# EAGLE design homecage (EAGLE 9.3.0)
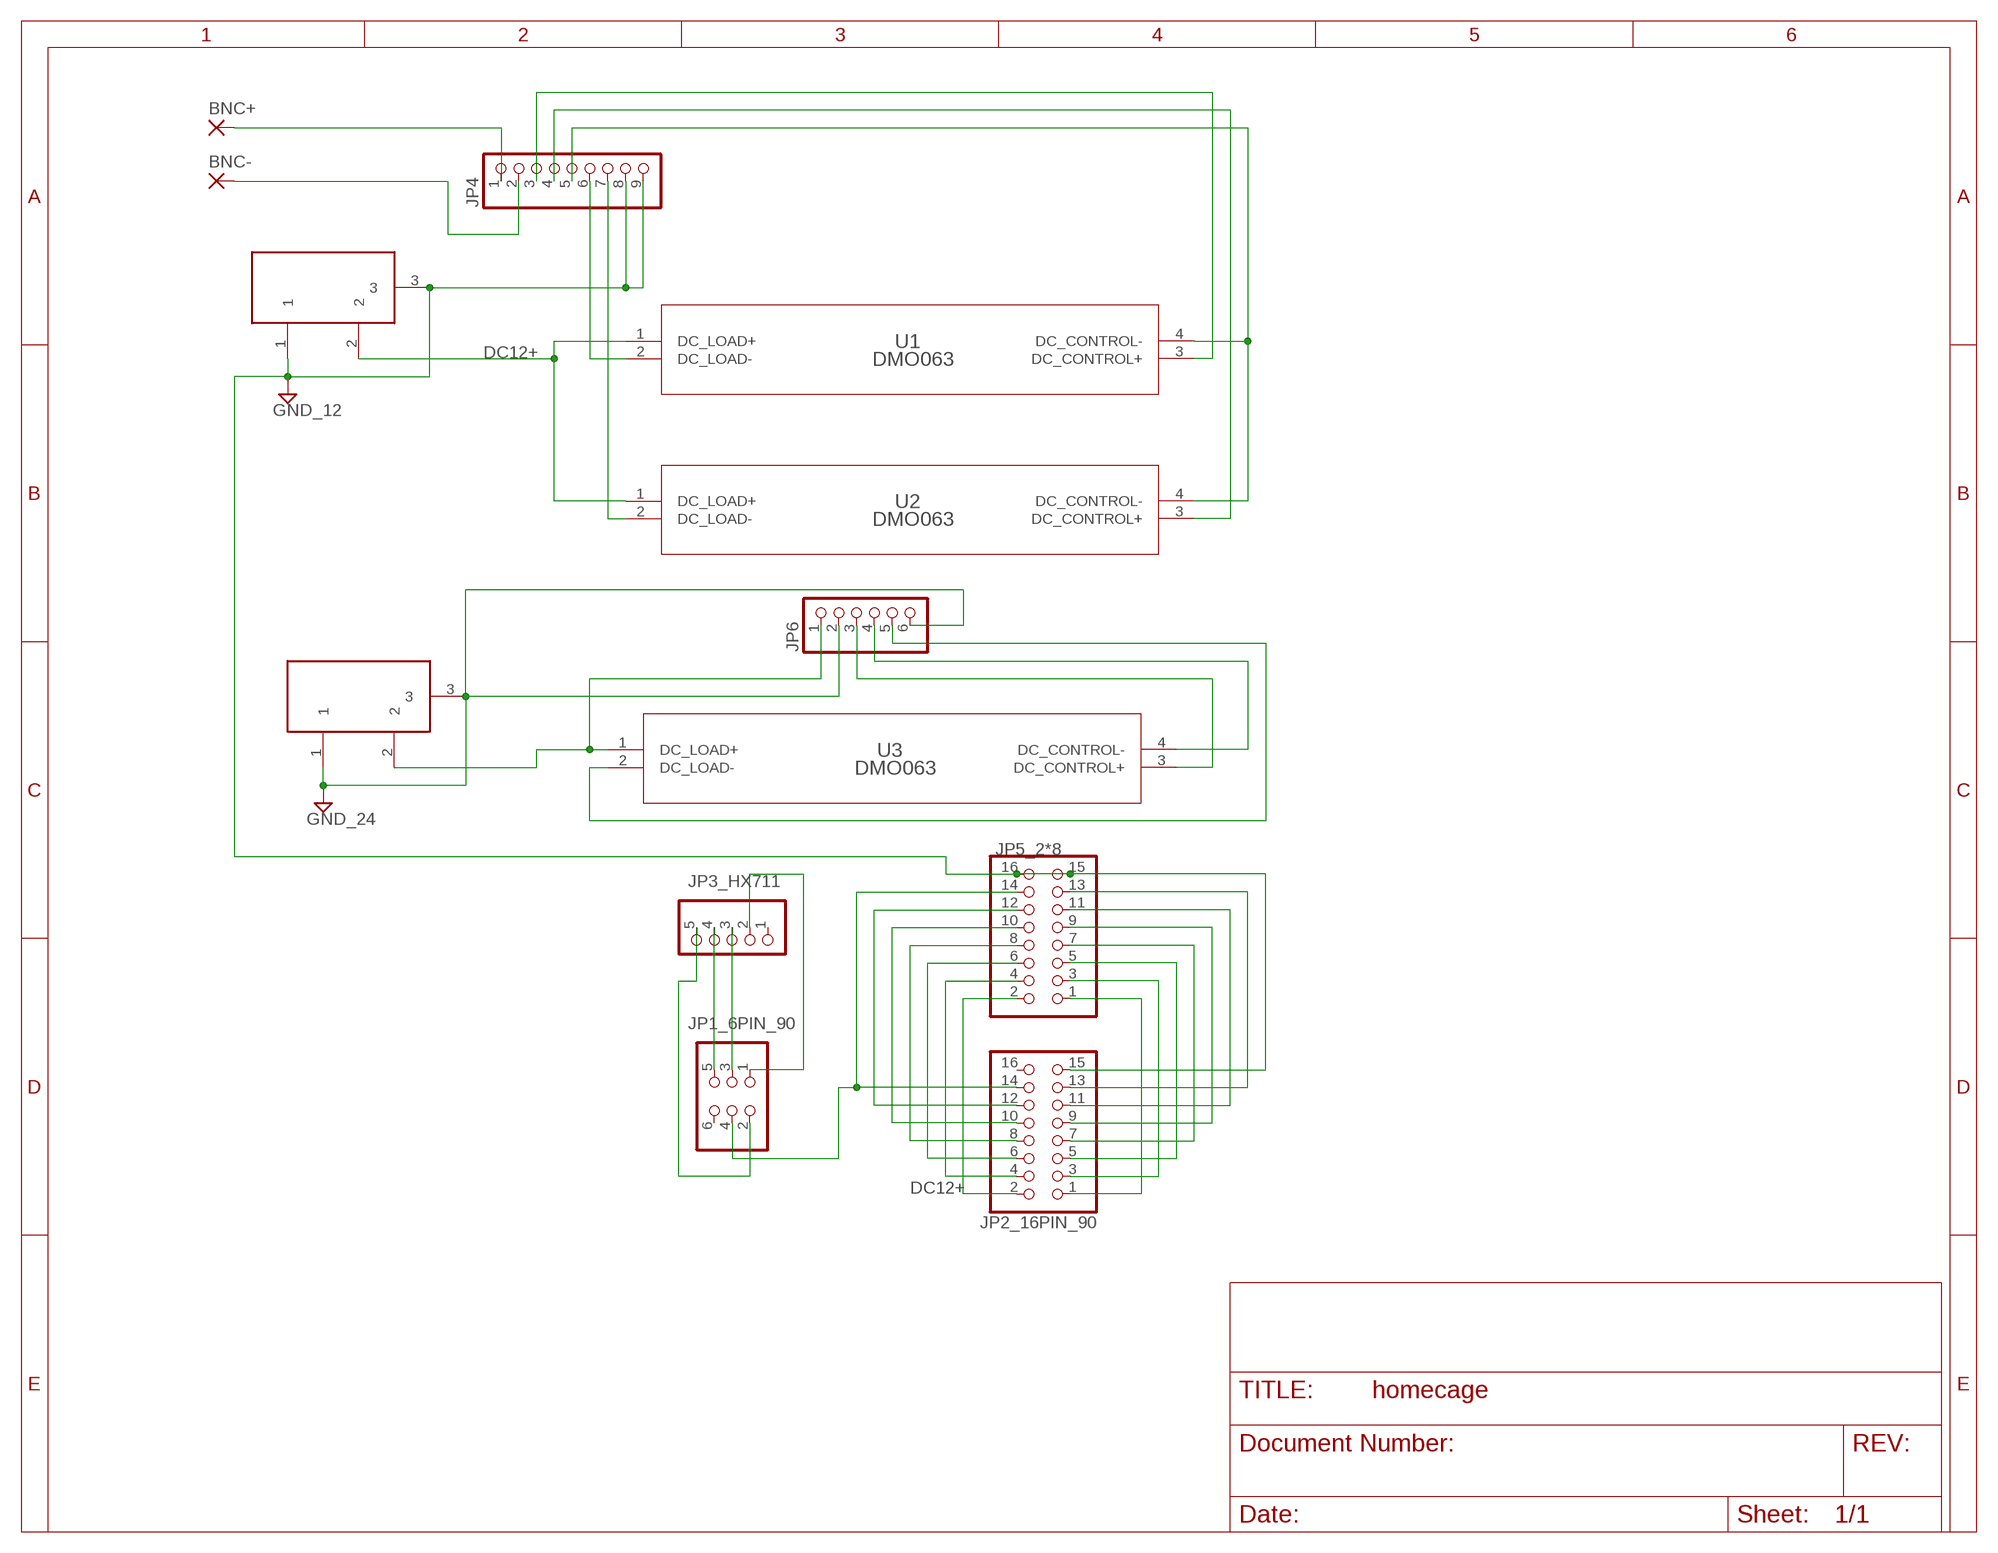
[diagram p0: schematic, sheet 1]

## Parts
BNC+  SMD5  [SMD2,54-5,08]
BNC-  SMD5  [SMD2,54-5,08]
DC12V  POWERSUPPLY_DC21MMX  [POWERSUPPLY_DC-21MM]
DC24V  POWERSUPPLY_DC21MMX  [POWERSUPPLY_DC-21MM]
JP1_6PIN_90  PINHD-2X3/90  [2X03/90]
JP2_16PIN_90  PINHD-2X8/90  [2X08/90]
JP3_HX711  PINHD-1X5  [1X05]
JP4  PINHD-1X9  [1X09]
JP5_2*8  PINHD-2X8  [2X08]
JP6  PINHD-1X6  [1X06]
U1  DMO063  [SIP-4_DMO]
U2  DMO063  [SIP-4_DMO]
U3  DMO063  [SIP-4_DMO]

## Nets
DC12+ [power]: DC12V.2 JP2_16PIN_90.2 JP5_2*8.2 U1.1(DC_LOAD+) U2.1(DC_LOAD+)
GND1 [power]: DC12V.1 DC12V.3 JP2_16PIN_90.15 JP4.8 JP4.9 JP5_2*8.15 JP5_2*8.16 ; supply symbol labelled GND_12
GND2 [power]: DC24V.1 DC24V.3 JP6.2 JP6.6 ; supply symbol labelled GND_24
N$1: JP2_16PIN_90.1 JP5_2*8.1
N$2: JP2_16PIN_90.3 JP5_2*8.3
N$3: JP2_16PIN_90.5 JP5_2*8.5
N$4: JP2_16PIN_90.7 JP5_2*8.7
N$5: JP2_16PIN_90.9 JP5_2*8.9
N$6: JP2_16PIN_90.11 JP5_2*8.11
N$7: JP2_16PIN_90.13 JP5_2*8.13
N$8: JP4.6 U1.2(DC_LOAD-)
N$10: JP2_16PIN_90.4 JP5_2*8.4
N$11: JP2_16PIN_90.6 JP5_2*8.6
N$12: JP2_16PIN_90.8 JP5_2*8.8
N$13: JP2_16PIN_90.10 JP5_2*8.10
N$14: JP2_16PIN_90.12 JP5_2*8.12
N$15: JP1_6PIN_90.4 JP2_16PIN_90.14 JP5_2*8.14
N$17: JP1_6PIN_90.1 JP3_HX711.2
N$18: JP1_6PIN_90.3 JP3_HX711.3
N$19: JP1_6PIN_90.5 JP3_HX711.4
N$20: JP1_6PIN_90.2 JP3_HX711.5
N$22 [power]: DC24V.2 JP6.1 U3.1(DC_LOAD+)
N$23: JP4.7 U2.2(DC_LOAD-)
N$24: JP4.5 U1.4(DC_CONTROL-) U2.4(DC_CONTROL-)
N$25: BNC+.1(P) JP4.1
N$26: JP4.4 U2.3(DC_CONTROL+)
N$27: JP4.3 U1.3(DC_CONTROL+)
N$28: BNC-.1(P) JP4.2
N$30: JP6.3 U3.3(DC_CONTROL+)
N$31: JP6.4 U3.4(DC_CONTROL-)
N$32: JP6.5 U3.2(DC_LOAD-)
Unconnected: JP1_6PIN_90.6 JP2_16PIN_90.16 JP3_HX711.1

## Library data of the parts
BNC+ BNC- = wirepad:SMD5: SMD PAD
DC12V DC24V = Arduino_MEGA2560_ref:POWERSUPPLY_DC21MM
JP1_6PIN_90 = pinhead:PINHD-2X3: PIN HEADER
JP2_16PIN_90 JP5_2*8 = pinhead:PINHD-2X8: PIN HEADER
JP3_HX711 = pinhead:PINHD-1X5: PIN HEADER
JP4 = pinhead:PINHD-1X9: PIN HEADER
JP6 = pinhead:PINHD-1X6: PIN HEADER
U1-U3 = homecage:DMO063; MANUFACTURER_PART_NUMBER: DMO063; VENDOR: Crydom

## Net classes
0 default: width 0.406 mm
1 power: width 1.219 mm

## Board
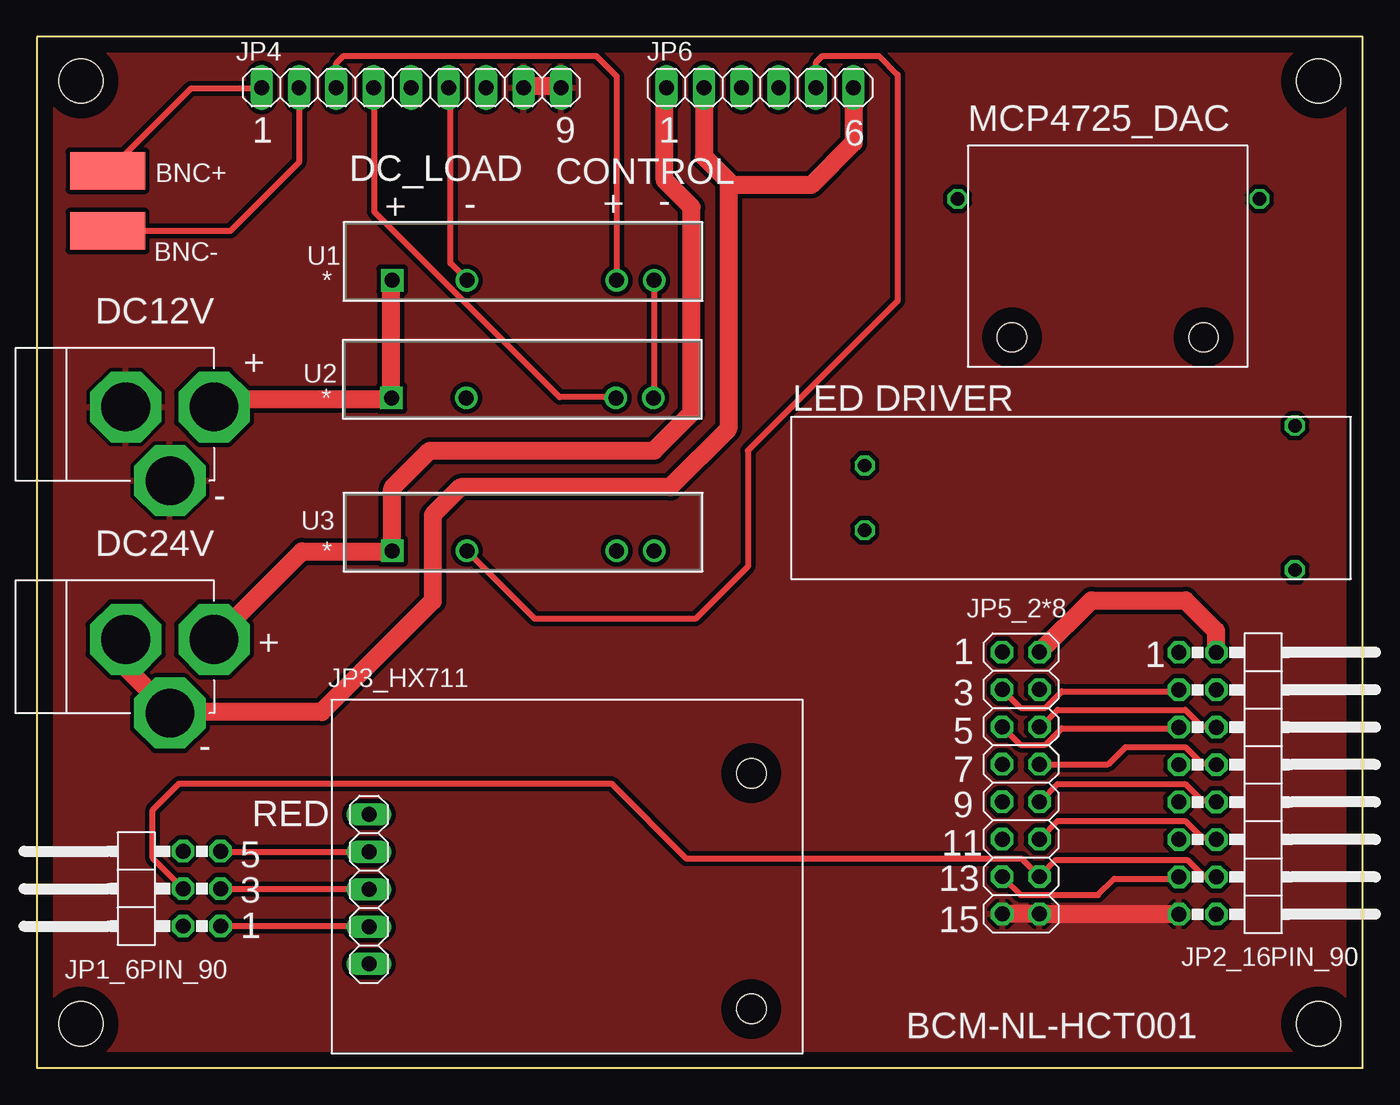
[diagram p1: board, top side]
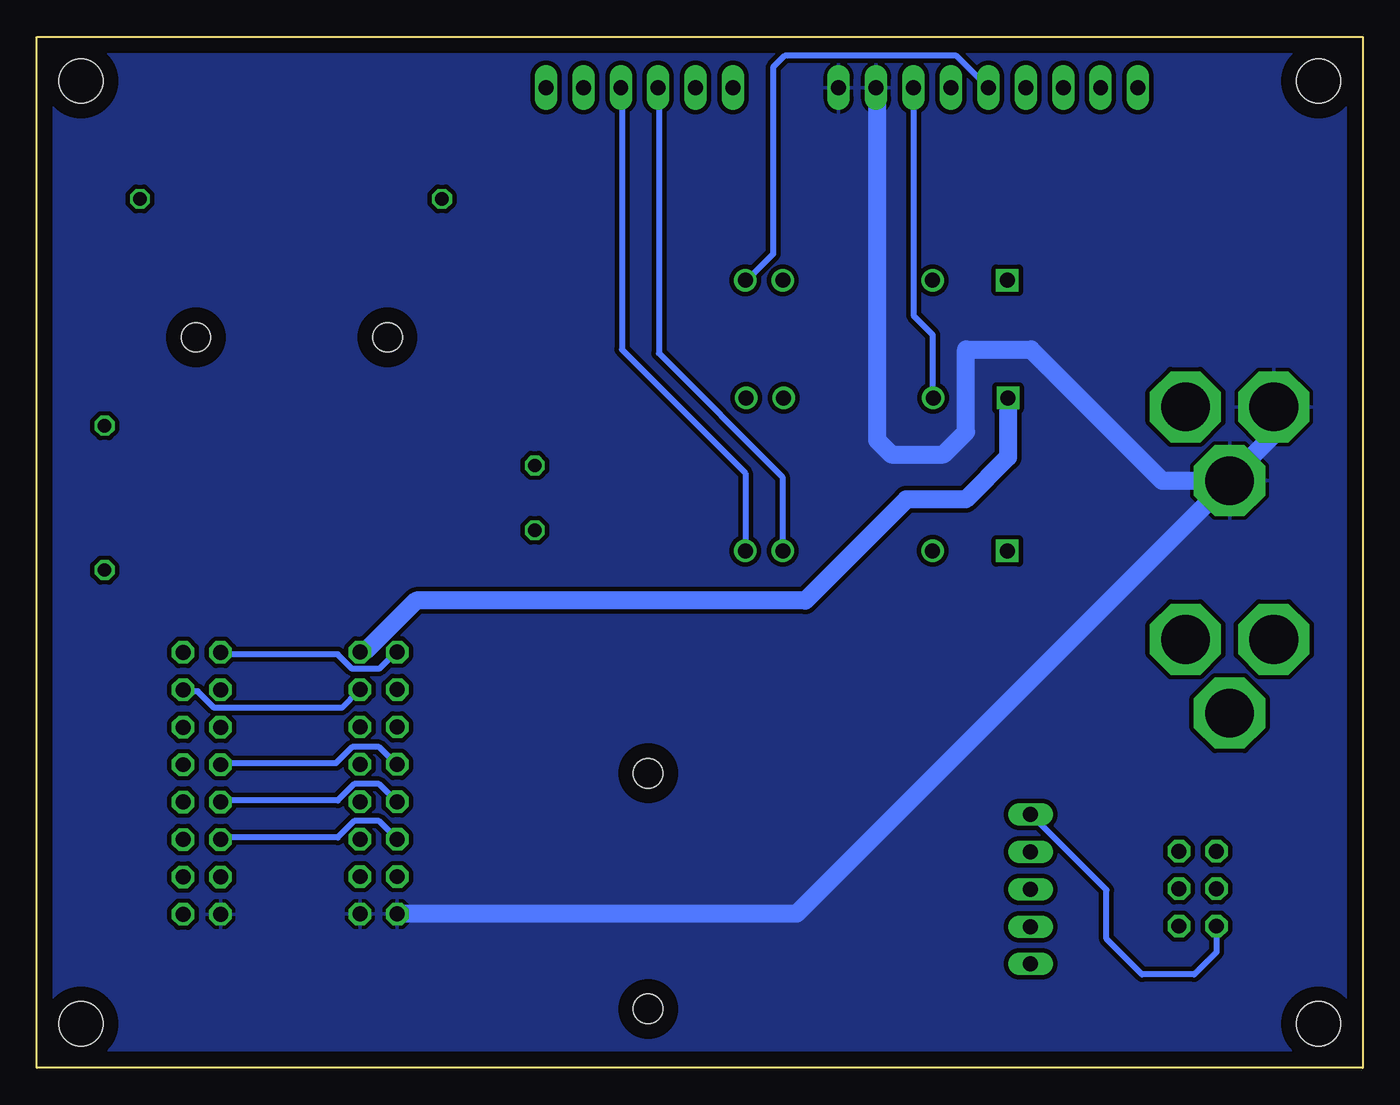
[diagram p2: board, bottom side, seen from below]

Size 90 x 70 mm. Coordinates in mm from the lower left corner, seen from the top.
Outline: 0,0 90,0 90,70 0,70 0,0
Copper layers (1*16): Top 0.035mm / dielectric 1.5mm / Bottom 0.035mm
Design rules "default": minimum track width 6mil, minimum drill 0.35mm, track to track 6mil, track to pad 6mil, pad to pad 6mil, via to via 6mil, smd to smd 6mil, copper to edge 40mil, drill to drill 6mil, minimum pad ring 10mil, minimum via ring 8mil, stop-mask expansion 4mil, vias tented up to drill 0mil, thermal gap 10mil
Holes 3 mm at 3,3 3,67 87,67 87,3
Holes 2 mm at 48.5,20 48.5,4 66.2,49.6 79.2,49.6

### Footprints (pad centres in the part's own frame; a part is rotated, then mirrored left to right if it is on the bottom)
SMD2,54-5,08 = smd 2.54 x 5.08: 1 0,0
POWERSUPPLY_DC-21MM = drill 3.302 pad 4.826 octagon: 1 -5.08,-3.353; 2 -0.076,-6.35; 3 -0.076,-0.356
2X03/90 = drill 1.016 octagon: 1 -2.54,-6.35; 2 -2.54,-3.81; 3 0,-6.35; 4 0,-3.81; 5 2.54,-6.35; 6 2.54,-3.81
2X08/90 = drill 1.016 octagon: 1 -8.89,-6.35; 2 -8.89,-3.81; 3 -6.35,-6.35; 4 -6.35,-3.81; 5 -3.81,-6.35; 6 -3.81,-3.81; 7 -1.27,-6.35; 8 -1.27,-3.81; 9 1.27,-6.35; 10 1.27,-3.81; 11 3.81,-6.35; 12 3.81,-3.81; 13 6.35,-6.35; 14 6.35,-3.81; 15 8.89,-6.35; 16 8.89,-3.81
1X05 = drill 1.016 long: 1 -5.08,0; 2 -2.54,0; 3 0,0; 4 2.54,0; 5 5.08,0
1X09 = drill 1.016 long: 1 -10.16,0; 2 -7.62,0; 3 -5.08,0; 4 -2.54,0; 5 0,0; 6 2.54,0; 7 5.08,0; 8 7.62,0; 9 10.16,0
2X08 = drill 1.016 octagon: 1 -8.89,-1.27; 2 -8.89,1.27; 3 -6.35,-1.27; 4 -6.35,1.27; 5 -3.81,-1.27; 6 -3.81,1.27; 7 -1.27,-1.27; 8 -1.27,1.27; 9 1.27,-1.27; 10 1.27,1.27; 11 3.81,-1.27; 12 3.81,1.27; 13 6.35,-1.27; 14 6.35,1.27; 15 8.89,-1.27; 16 8.89,1.27
1X06 = drill 1.016 long: 1 -6.35,0; 2 -3.81,0; 3 -1.27,0; 4 1.27,0; 5 3.81,0; 6 6.35,0
SIP-4_DMO = drill 1.016 pad 1.524 square: 1 -17.78,-2.54 | drill 1.016 pad 1.524: 2 -12.7,-2.54; 3 -2.54,-2.54; 4 0,-2.54

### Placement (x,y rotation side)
BNC+  4.8,60.9 90 top
BNC-  4.8,56.82 90 top
DC12V  5.68,44.95 90 top
DC24V  5.68,29.17 90 top
JP1_6PIN_90  6.12,12.17 90 top
JP2_16PIN_90  83.88,19.32 270 top
JP3_HX711  22.55,12.13 90 top
JP4  25.41,66.55 0 top
JP5_2*8  66.8,19.34 270 top
JP6  49.09,66.55 0 top
U1  41.9,56.02 0 top
U2  41.85,48.02 0 top
U3  41.9,37.64 0 top

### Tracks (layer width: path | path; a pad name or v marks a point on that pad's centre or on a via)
DC12+
  Top 1.219: JP2_16PIN_90.2 80.05,28.22 80.05,29.68 77.98,31.75 71.59,31.75 JP5_2*8.2 | U1.1 24.03,53.37 24.03,45.54 U2.1 23.47,45.4 12.57,45.4 12.15,44.98 DC12V.2
  Bottom 1.219: JP5_2*8.2 68.03,28.36 67.61,28.36 64.24,31.73 37.84,31.73 30.98,38.59 26.94,38.59 24.07,41.46 U2.1
GND1
  Top 1.219: JP5_2*8.15 65.66,10.48 68.03,10.48 JP5_2*8.16 68.59,10.48 77.39,10.48 JP2_16PIN_90.15 | JP4.8 33.11,66.64 35.48,66.64 JP4.9
  Bottom 1.219: JP4.8 32.97,66.5 32.97,42.62 32,41.66 28.45,41.66 26.92,43.18 26.92,48.77 22.52,48.77 13.62,39.87 DC12V.1 | JP5_2*8.15 65.52,10.48 38.42,10.48 DC12V.1 | DC12V.3 6.15,44.84 6.15,42.89 8.66,40.37 DC12V.1
  pour Top (isolate 0.305): 0,0 0,70 90,70 90,0
  pour Bottom (isolate 0.305): 0,0 0,70 90,70 90,0
  pour Top (isolate 0.305): 0,0 0,70 90,70 90,0
GND2
  Top 1.219: 45.4,65.94 45.4,66.5 JP6.2 45.28,61.86 46.94,60.2 | 55.32,65.94 55.32,66.5 JP6.6 55.44,62.81 52.58,59.94 47.19,59.94 46.94,60.2 | DC24V.3 6.15,29.06 6.15,27.1 8.66,24.59 DC24V.1 9.08,24.17 19.34,24.17 26.87,31.69 26.87,37.53 28.77,39.43 42.99,39.43 46.94,43.38 46.94,60.2
N$1
  Bottom 0.406: JP2_16PIN_90.1 77.39,28.08 69.57,28.08 68.59,27.1 66.78,27.1 65.66,28.22 JP5_2*8.1
N$2
  Top 0.406: JP2_16PIN_90.3 77.39,25.57 69.57,25.57 68.45,24.45 66.78,24.45 65.66,25.57 JP5_2*8.3
N$3
  Top 0.406: JP2_16PIN_90.5 77.39,23.05 69.57,23.05 68.45,21.93 66.78,21.93 65.66,23.05 JP5_2*8.5
N$4
  Bottom 0.406: JP2_16PIN_90.7 77.39,20.68 69.71,20.68 68.59,21.79 66.78,21.79 65.66,20.68 JP5_2*8.7
N$5
  Bottom 0.406: JP2_16PIN_90.9 77.39,18.16 69.57,18.16 68.45,19.28 66.78,19.28 65.66,18.16 JP5_2*8.9
N$6
  Bottom 0.406: JP2_16PIN_90.11 77.39,15.65 69.57,15.65 68.45,16.76 66.78,16.76 65.66,15.65 JP5_2*8.11
N$7
  Top 0.406: JP2_16PIN_90.13 77.39,12.85 73.15,12.85 72.03,11.73 66.78,11.73 65.66,12.85 JP5_2*8.13
N$8
  Top 0.406: JP4.6 28.08,66.5 28.08,54.62 29.2,53.51 U1.2
N$9  (via drill 0.9 pad 1.3)
  other vias: 56.2,36.5
N$10
  Bottom 0.406: JP2_16PIN_90.4 80.05,25.57 79.07,25.57 77.95,24.45 69.29,24.45 68.17,25.57 JP5_2*8.4
N$11
  Top 0.406: JP2_16PIN_90.6 80.05,23.19 79.07,23.19 77.95,24.31 69.29,24.31 68.17,23.19 JP5_2*8.6
N$12
  Top 0.406: JP2_16PIN_90.8 80.05,20.68 79.07,20.68 77.95,21.79 73.91,21.79 72.73,20.61 JP5_2*8.8
N$13
  Top 0.406: JP2_16PIN_90.10 80.05,18.16 79.07,18.16 77.95,19.28 69.29,19.28 68.17,18.16 JP5_2*8.10
N$14
  Top 0.406: JP2_16PIN_90.12 80.05,15.65 79.07,15.65 77.95,16.76 69.29,16.76 68.17,15.65 JP5_2*8.12
N$15
  Top 0.406: JP2_16PIN_90.14 80.05,12.99 79.21,12.99 78.09,14.11 69.15,14.11 68.17,13.13 JP5_2*8.14 66.84,14.22 44.08,14.22 39,19.3 9.65,19.3 7.87,17.53 7.87,14.23 JP1_6PIN_90.4
N$16  (via drill 0.9 pad 1.3)
  other vias: 56.2,40.9
N$17
  Top 0.406: JP3_HX711.2 22.49,9.64 12.57,9.64 JP1_6PIN_90.1
N$18
  Top 0.406: JP3_HX711.3 22.49,12.15 12.57,12.15 JP1_6PIN_90.3
N$19
  Top 0.406: JP3_HX711.4 22.49,14.67 12.57,14.67 JP1_6PIN_90.5
N$20
  Bottom 0.406: JP3_HX711.5 22.49,17.18 17.39,12.08 17.39,8.75 14.99,6.35 11.43,6.35 9.93,7.85 JP1_6PIN_90.2
N$21  (via drill 0.9 pad 1.3)
  other vias: 85.4,43.6
N$22
  Top 0.406: 24.03,35.06 U3.1 | 42.61,66.5 JP6.1
  Top 1.219: DC24V.2 18,35.06 24.03,35.06 | U3.1 24.12,39.36 26.67,41.91 41.91,41.91 44.45,44.45 44.45,58.42 42.61,60.26 42.61,66.5
N$23
  Bottom 0.406: U2.2 29.2,45.54 29.2,49.78 30.49,51.08 JP4.7
N$24
  Top 0.406: U2.4 41.91,45.54 41.91,53.37 U1.4
  Bottom 0.406: U1.4 41.77,53.51 40.02,55.26 40.02,67.93 39.24,68.7 27.57,68.7 JP4.5
N$25
  Top 0.406: JP4.1 15.23,66.5 10.48,66.5 4.89,60.91 BNC+.1
N$26
  Top 0.406: U2.3 39.26,45.54 35.48,45.54 22.91,58.12 22.91,66.51 JP4.4
N$27
  Top 0.406: U1.3 39.36,67.32 37.98,68.7 20.83,68.7 20.33,68.21 JP4.3
N$28
  Top 0.406: JP4.2 17.79,61.48 13.13,56.82 BNC-.1
N$29  (via drill 0.9 pad 1.3)
  other vias: 85.4,33.8
N$30
  Bottom 0.406: U3.3 39.4,35.2 39.4,40.13 47.78,48.51 47.78,66.5 JP6.3
N$31
  Bottom 0.406: U3.4 41.91,35.2 41.91,40.39 50.29,48.77 50.29,66.5 JP6.4
N$32
  Top 0.406: JP6.5 52.9,68.27 53.34,68.7 57.15,68.7 58.42,67.44 58.42,52.07 48.26,41.91 48.26,34.04 44.7,30.48 33.82,30.48 U3.2
N$33  (via drill 0.9 pad 1.3)
  other vias: 83,59
N$34  (via drill 0.9 pad 1.3)
  other vias: 62.5,59

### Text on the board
tPlace: MCP4725_DAC | 1 | 9 | 1 | 6 | DC_LOAD | CONTROL | + | - | + | - | + | LED DRIVER | - | + | 1 | 1 | 3 | 5 | - | 7 | 9 | RED | 5 | 11 | 13 | 3 | 1 | 15 | BCM-NL-HCT001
